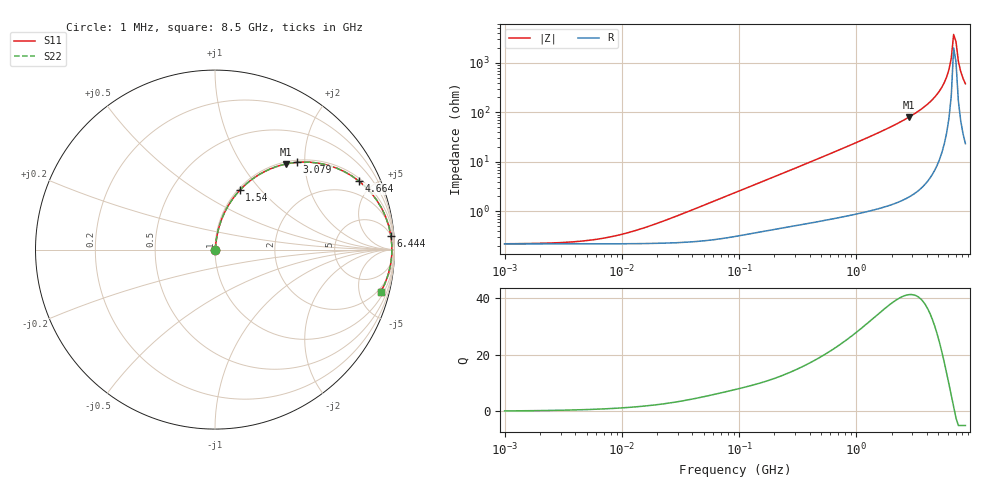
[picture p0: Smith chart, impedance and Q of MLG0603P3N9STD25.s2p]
! S-Parameter Data Generated by TDK Corporation
! Copyright(C) 2025 TDK Corporation.
! All Rights Reserved.
! TDK P/N: MLG0603P3N9STD25 (SMD / SMT Inductor (Coil))
! Property: L=3.9nH at 500MHz
! Size(LxWxT): 0.6x0.3x0.3mm
! Model Type: s2p (Touchstone File Format Version 1.0)
! Frequency: DC=Yes Start=1MHz Stop=8500MHz 198points Log-sweep
! Model Generated on Feb. 6, 2025
! Terms and conditions regarding TDK Simulation Models:
! 1)This simulation model is being provided solely for informational
!  purposes. Please refer to the specifications of the products in
!  terms of detailed characteristics of such products.
! 2)In no event shall TDK Corporation of any of its subsidiaries be
!  liable for any loss or damage arising, directly or indirectly,
!  from any information contained in this simulation model, including,
!  but not limited to loss or damages arising from any inaccuracies,
!  omissions or errors in connection with such information.
! 3)Any and all copyrights on this simulation model are owned by
!  TDK Corporation.  Duplication or redistribution of this simulation
!  model without prior written permission from TDK Corporation
!  is prohibited.
! 4)This simulation model is subject to any modification or change
!  without any prior notice.
! 5)Neither TDK Corporation nor any of its subsidiaries shall make any
!  warranty, express or implied, including but not limited to the
!  correctness, implied warranties of merchantability and fitness for
!  a particular purpose with respect to this simulation models.
! 6)The use of this simulation model shall be deemed to have consented
!  to the terms and conditions hereof.
! Port Assignments:
!  1 ---@@@--- 2
! Applicable Conditions:
!  Temperature = 25 degC
!  DC Bias Current = 0 A
!  Small Signal Operation
# Hz S MA R 50
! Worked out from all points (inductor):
!   197 points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, 1 MHz to 8.5 GHz, reference 50 ohm
!   read as one part in series: L = 4.18 nH near 26.51 MHz
!   highest Q = 41.1 at 2.807 GHz (marker M1), where L = 4.54 nH
!   self-resonance near 6.748 GHz
!   S11 on the Smith chart (normalised r, x): 1 MHz: 1.00, +0.00; 1.54 GHz: 1.02, +0.78; 3.079 GHz: 1.04, +1.83; 4.664 GHz: 1.14, +4.10; 6.444 GHz: 5, +24; 8.5 GHz: 1.47, -7.57
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1000000  0.002211 6.8  0.9978 -0.0  0.9978 -0.0  0.002211 6.8
4587603  0.002508 28.7  0.9978 -0.1  0.9978 -0.1  0.002508 28.7
9601846  0.003356 48.7  0.9978 -0.1  0.9978 -0.1  0.003356 48.7
2.10461e7  0.005974 67.4  0.9977 -0.3  0.9977 -0.3  0.005974 67.4
9.219544e7  0.02385 81.2  0.9966 -1.4  0.9966 -1.4  0.02385 81.2
4.229561e8  0.1029 80.8  0.9889 -5.9  0.9889 -5.9  0.1029 80.8
9.270694e8  0.2202 75.1  0.9673 -12.7  0.9673 -12.7  0.2202 75.1
1.540426e9  0.3584 67.3  0.9232 -21.0  0.9232 -21.0  0.3584 67.3
1.940355e9  0.4449 62.1  0.8839 -26.4  0.8839 -26.4  0.4449 62.1
2.80715e9  0.6181 50.4  0.7712 -38.2  0.7712 -38.2  0.6181 50.4
3.07866e9  0.6672 46.8  0.7288 -41.8  0.7288 -41.8  0.6672 46.8
3.877948e9  0.7936 36.0  0.5877 -52.5  0.5877 -52.5  0.7936 36.0
4.664383e9  0.8871 25.6  0.4328 -62.5  0.4328 -62.5  0.8871 25.6
5.115526e9  0.9261 19.9  0.3409 -67.7  0.3409 -67.7  0.9261 19.9
5.610304e9  0.9569 13.9  0.2406 -72.8  0.2406 -72.8  0.9569 13.9
6.152938e9  0.9773 7.7  0.1339 -76.4  0.1339 -76.4  0.9773 7.7
6.44363e9  0.983 4.5  0.0792 -75.4  0.0792 -75.4  0.983 4.5
6.748056e9  0.9857 1.3  0.02628 -56.5  0.02628 -56.5  0.9857 1.3
7.066863e9  0.9852 -1.9  0.03656 65.2  0.03656 65.2  0.9852 -1.9
7.400733e9  0.9816 -5.1  0.09051 75.7  0.09051 75.7  0.9816 -5.1
7.750377e9  0.9748 -8.3  0.1451 75.9  0.1451 75.9  0.9748 -8.3
8.5e9  0.9526 -14.5  0.2512 71.9  0.2512 71.9  0.9526 -14.5
